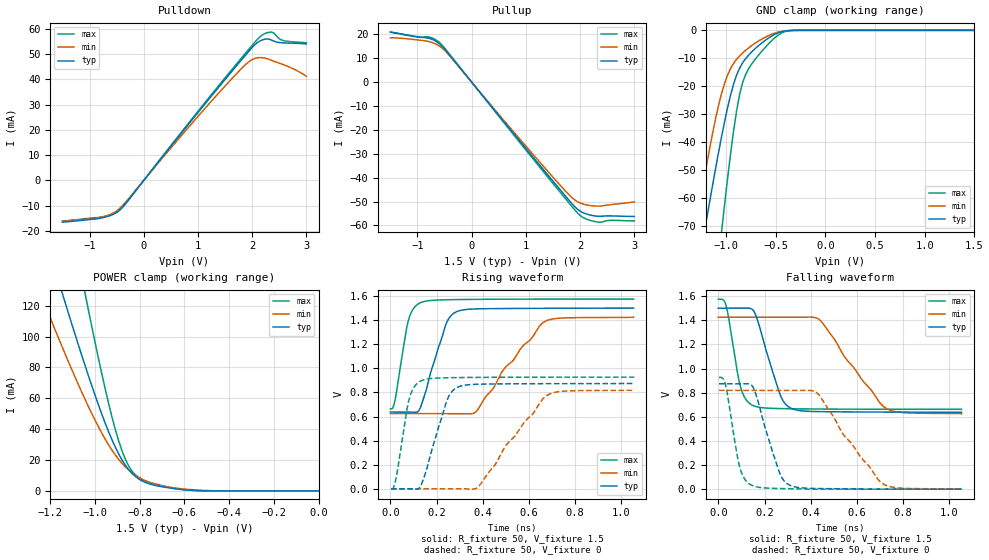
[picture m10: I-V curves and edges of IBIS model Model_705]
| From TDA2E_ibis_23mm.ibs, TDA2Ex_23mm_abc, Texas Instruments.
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| Model based on original model for DDR_DIFFIOPB_V
|   Sub model SR000_DRV34_1P5
[model]   Model_705
|[Description]  [1.5V-I/O-X-X]
|   , ,
|[Input Load]
|[Output Drive]
|Voltage   1.5V
|Mode   I/O
Model_type   I/O
Polarity   Non-Inverting
Enable   Active-Low
Vinl =  0.65
Vinh =  0.85
Cref =  15.0000pF
Rref =  100.0000M
Vref =  0V
Vmeas =  0.75
C_comp   2p   2p   2p
[Model Spec]
Vinl   0.65   0.6125   0.6875
Vinh   0.85   0.8125   0.8875
[Receiver Thresholds]
Tslew_ac = 0.5n
Vth= 0.75
Vth_max= 0.7875
Vth_min= 0.675
Vinh_ac= 0.175
Vinh_dc= 0.1
Vinl_ac= -0.175
Vinl_dc= -0.1
[Temperature Range]   25   125   -40
[Voltage Range]   1.5   1.425   1.575
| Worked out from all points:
|   slope of the pulldown table from 0 to 0.225 V, typ, clamps not added: 36.8 ohm
|   slope of the pullup table from 0 to 0.225 V, typ, clamps not added: 35.8 ohm
|   GND clamp passes 1 mA (typ) near -0.48 V on its own axis
|   POWER clamp passes 1 mA (typ) near -0.62 V on its own axis
|   rising waveform, R_fixture 50, V_fixture 1.5: 20-80 % time 80.3ps typ, 195ps min, 47.3ps max; typ from 0.637 V to 1.5 V
|   rising waveform, R_fixture 50, V_fixture 0: 20-80 % time 80ps typ, 190ps min, 47.6ps max; typ from 0 V to 0.874 V
|   falling waveform, R_fixture 50, V_fixture 1.5: 20-80 % time 81.3ps typ, 181ps min, 49.7ps max; typ from 1.5 V to 0.637 V
|   falling waveform, R_fixture 50, V_fixture 0: 20-80 % time 81.2ps typ, 183ps min, 49ps max; typ from 0.874 V to 0 V
[POWER_clamp]
-1.5V     302.8mA    223.9mA    484.4mA
-1.242V   174.3mA    127.3mA    279.1mA
-1.136V   123.3mA    89.68mA    196.8mA
-1.045V   81.65mA    59.62mA    128.8mA
-1.03V    75mA       54.92mA    117.8mA
-939.4mV  38.44mA    29.91mA    56.84mA
-893.9mV  23.93mA    20.41mA    32.31mA
-848.5mV  13.61mA    13.43mA    15.91mA
-803mV    7.623mA    8.663mA    8.564mA
-712.1mV  3.022mA    3.561mA    3.877mA
-575.8mV  470.5uA    872uA      449uA
0V        112.6nA    435.6nA    613.8nA
[Pulldown]
-1.5V     -16.54mA   -16.32mA   -16.11mA
-727.3mV  -14.62mA   -14.26mA   -14.29mA
-545.5mV  -13.24mA   -12.72mA   -13.05mA
-409.1mV  -10.94mA   -10.36mA   -11.07mA
1.227V    32.84mA    30.87mA    33.41mA
1.818V    48.09mA    44.61mA    48.84mA
2V        52.62mA    47.82mA    53.46mA
2.182V    55.55mA    48.58mA    57.5mA
2.273V    55.99mA    48.2mA     58.42mA
2.364V    55.5mA     47.46mA    58.71mA
2.545V    54.48mA    46.06mA    55.55mA
3V        54mA       41.23mA    54.49mA
[Pullup]
-1.5V     20.96mA    18.6mA     20.95mA
-1V       19mA       17.69mA    18.93mA
-772.7mV  18.26mA    16.89mA    18.84mA
-590.9mV  16.04mA    15.07mA    16.54mA
-409.1mV  11.43mA    11.07mA    11.7mA
1.409V    -38.97mA   -37.46mA   -39.88mA
1.773V    -48.83mA   -46.66mA   -49.96mA
1.909V    -52.33mA   -49.44mA   -53.68mA
2.045V    -54.57mA   -50.97mA   -56.55mA
2.273V    -56.03mA   -51.89mA   -58.38mA
2.591V    -56.03mA   -51.23mA   -57.86mA
3V        -56.26mA   -50.14mA   -58.12mA
[GND_clamp]
-1.5V     -133.6mA   -115.7mA   -234.3mA
-1.288V   -87.29mA   -67.59mA   -156.8mA
-1.197V   -68.11mA   -48.64mA   -124.4mA
-1.045V   -38.25mA   -22.77mA   -72.51mA
-1.015V   -32.88mA   -19.1mA    -62.74mA
-954.5mV  -23.3mA    -13.72mA   -44.4mA
-863.6mV  -13.6mA    -9.192mA   -23.11mA
-803mV    -10.18mA   -7.193mA   -15.89mA
-681.8mV  -5.771mA   -4.027mA   -9.287mA
-500mV    -1.264mA   -914.7uA   -2.429mA
-348.5mV  -52.39uA   -75.11uA   -85.87uA
1.5V      112.6nA    528.1nA    514.5nA
[Ramp]
dV/dt_f 0.51822039/81.426924p 0.48131424/0.18143951n 0.54809572/49.733101p
dV/dt_r 0.52638885/80.290439p 0.49338698/0.19127697n 0.55808744/47.754238p
R_load = 50
[Rising Waveform]
R_fixture = 50
V_fixture = 1.5
V_fixture_min = 1.425
V_fixture_max = 1.575
0s        637.3mV    624.3mV    662.9mV
20.34ps   636.6mV    624.2mV    737.5mV
78.04ps   636.6mV    624.2mV    1.398V
129.3ps   671.4mV    624.2mV    1.544V
240ps     1.362V     624mV      1.569V
285.2ps   1.469V     623.6mV    1.571V
371ps     1.493V     640.8mV    1.573V
491ps     1.497V     993.1mV    1.574V
670.1ps   1.498V     1.39V      1.575V
1.053ns   1.5V       1.425V     1.575V
[Rising Waveform]
R_fixture = 50
V_fixture = 0
V_fixture_min = 0
V_fixture_max = 0
2.917ps   0V         0V         0V
24.43ps   0V         0V         83.95mV
82.3ps    0V         0V         750.8mV
134.2ps   36.56mV    0V         897.5mV
244.6ps   731.7mV    0V         921.7mV
290.6ps   842.8mV    0V         923.2mV
382ps     868.2mV    19.63mV    924.8mV
501.6ps   871.1mV    363mV      925.9mV
680.9ps   872.7mV    778.5mV    926.5mV
1.056ns   874.1mV    819mV      926.7mV
[Falling Waveform]
R_fixture = 50
V_fixture = 1.5
V_fixture_min = 1.425
V_fixture_max = 1.575
0s        1.5V       1.425V     1.575V
35.51ps   1.5V       1.425V     1.509V
83.38ps   1.5V       1.425V     962.4mV
100.5ps   1.5V       1.425V     820.7mV
148.5ps   1.488V     1.425V     695mV
268.5ps   779.7mV    1.425V     667.9mV
313.2ps   672.1mV    1.425V     666.4mV
442.3ps   642.6mV    1.397V     664mV
729.5ps   638.8mV    666.3mV    662.5mV
1.053ns   637.3mV    624.3mV    662.3mV
[Falling Waveform]
R_fixture = 50
V_fixture = 0
V_fixture_min = 0
V_fixture_max = 0
2.917ps   874.1mV    819mV      926.7mV
33.06ps   874.3mV    819.1mV    852.5mV
95.54ps   873.6mV    819.1mV    164.2mV
145.9ps   858mV      819.1mV    31.04mV
263.7ps   141.3mV    819.1mV    5.241mV
309.4ps   32.86mV    818.8mV    3.552mV
431.6ps   5.313mV    790mV      0V
540.9ps   2.955mV    454.1mV    0V
714.7ps   0V         41.84mV    0V
1.056ns   0V         0V         0V
